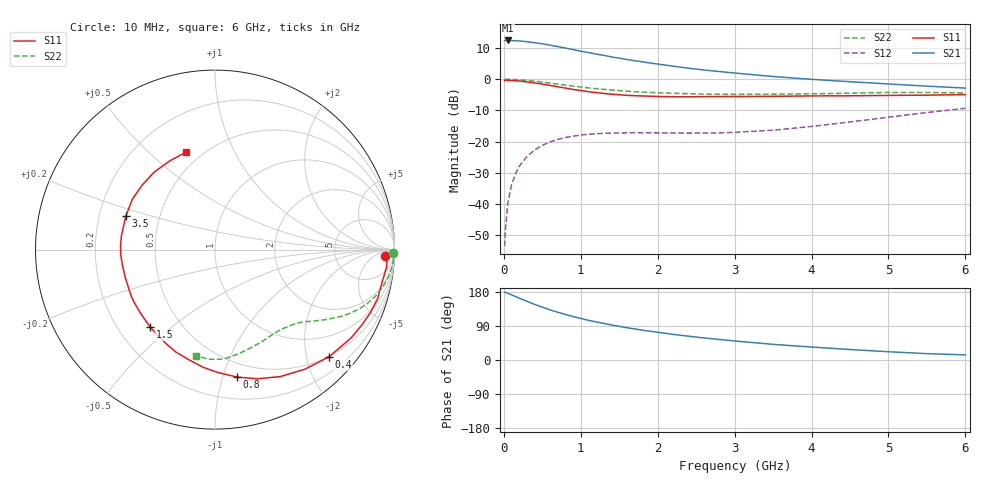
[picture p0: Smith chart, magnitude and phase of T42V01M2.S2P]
! Infineon Technologies  Discrete & RF Semiconductors
! BFR182T
! Si NPN RF Bipolar Junction Transistor in SC75
! VCE = 2 V  IC = 1.2 mA
! Common Emitter S-Parameters:  October  1999
# GHz  S  MA  R  50
!  f  S11  S21  S12  S22
! GHz  MAG  ANG  MAG  ANG  MAG  ANG  MAG  ANG
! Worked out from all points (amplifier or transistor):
!   36 points, 10 MHz to 6 GHz, reference 50 ohm
!   highest |S21| = 12.4 dB at 50 MHz (marker M1)
!   |S21| within 3 dB of that: start of sweep to 911.3 MHz
!   unconditionally stable (mu >= 1): 2.273 GHz to 4.547 GHz
!   at 250 MHz: K = 0.11, MSG = 19.2 dB, |S12| = -26.3 dB
!   at 1.4 GHz: K = 0.64, MSG = 12.2 dB, |S12| = -17.3 dB
!   at 6 GHz: K = 0.84, MSG = 3.2 dB, |S12| = -9.3 dB
!   S11 on the Smith chart (normalised r, x): 10 MHz: 24, -17; 400 MHz: 0.49, -2.44; 800 MHz: 0.38, -1.12; 1.5 GHz: 0.34, -0.42; 3.5 GHz: 0.32, +0.16; 6 GHz: 0.41, +0.66
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0.01  0.9465 -2.2  4.153 178.6  0.0021 88.1  0.9923 -1.2
0.02  0.9575 -0.8  4.164 178.8  0.0038 102.9  0.9889 -0.8
0.05  0.9612 -5.7  4.18 175.8  0.0099 90.0  0.9966 -2.3
0.1  0.9487 -10.8  4.157 172.0  0.0203 83.5  0.9936 -4.4
0.15  0.9463 -16.9  4.143 167.4  0.0301 79.1  0.9859 -6.6
0.25  0.9197 -27.2  4.049 159.1  0.0484 74.0  0.9681 -10.8
0.3  0.9041 -32.9  3.991 154.9  0.0574 71.4  0.9571 -12.7
0.4  0.8724 -43.2  3.851 146.7  0.0732 65.4  0.9286 -16.5
0.5  0.8339 -53.0  3.688 139.5  0.0865 60.3  0.8982 -19.7
0.6  0.7956 -62.8  3.513 132.3  0.0987 55.6  0.8657 -22.6
0.8  0.721 -80.1  3.162 120.1  0.1161 48.0  0.8037 -27.4
0.9  0.6845 -88.8  2.979 114.6  0.122 44.7  0.7743 -29.2
1.1  0.6299 -103.6  2.673 104.7  0.1309 39.8  0.7267 -32.5
1.3  0.5906 -117.4  2.411 96.4  0.136 36.1  0.6863 -35.3
1.5  0.563 -129.8  2.173 88.8  0.1373 33.7  0.6577 -37.5
1.8  0.5382 -146.4  1.901 78.7  0.1381 31.9  0.6205 -41.1
2.2  0.5235 -163.0  1.618 67.7  0.1374 32.6  0.5948 -45.6
2.8  0.5267 177.4  1.327 54.2  0.1376 38.1  0.5725 -53.6
3.5  0.5309 159.4  1.104 41.3  0.152 47.9  0.5756 -63.1
4.5  0.542 138.7  0.911 27.7  0.2062 57.7  0.5964 -78.0
5.5  0.5547 117.0  0.774 16.8  0.292 58.1  0.6119 -92.9
6  0.5664 106.7  0.72 13.5  0.3413 55.4  0.6023 -99.9
